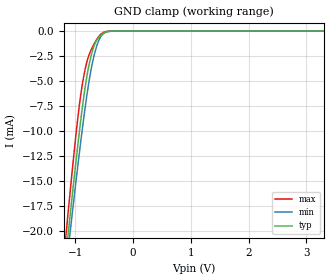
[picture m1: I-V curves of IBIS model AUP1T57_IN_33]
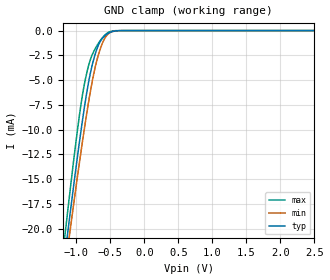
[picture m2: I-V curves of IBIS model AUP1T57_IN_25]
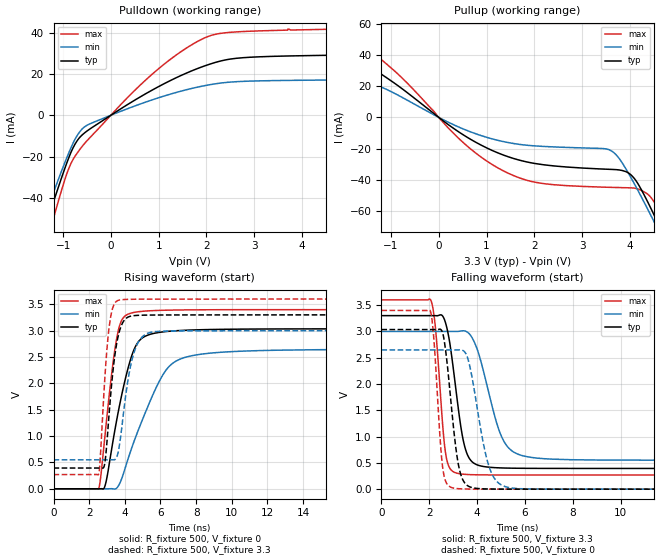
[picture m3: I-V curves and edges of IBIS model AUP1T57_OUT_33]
| TEXAS INSTRUMENTS INCORPORATED
| Standard Linear and Logic Group
| IBIS Model of SN74AUP1T57
| SINGLE-SUPPLY VOLTAGE TRANSLATER
| This file contains package information for the following:
|  SOT 6-pin (DBV) package as [Component] AUP1T57_DBV
|  SOT 6-pin (DCK) package as [Component] AUP1T57
|  DSBGA 6-pin (YEP_YZP) package as [Component] AUP1T57_YEP_YZP
| This device can be powered at the following Vccs:
|  3.3 volt Vcc
|  2.5 volt Vcc
| This file provides unique models under the [Model Selector] for each Vcc.
| For operation at a specific Vcc, select the appropriate model after each
| [Model Selector] keyword.
[IBIS Ver]   3.2
[Comment char]  |_char
[File Name]   sn74aup1t57.ibs
[File Rev]   1.1 | x_die
[Date]   July 14, 2004
[Source]   Data created from TI-SPICE simulations at TI-SLL.
[Notes]   The following is an IBIS list for the AUP1T57.
   Please contact sllibis@ti.com with questions and
   comments concerning SLL IBIS models.
   - FILE REV HISTORY
   - 1.1 Release IBIS file on 10/01/04
   - Non-monotonic data in pullup due to special output circuit.
   - Power clamp data deleted as there is no power-clamp diode.
   - YEP and YZP packages are package preview only at this date.
[Disclaimer] Property of Texas Instruments Incorporated.  Unauthorized
   reproduction and/or distribution is strictly prohibited.
   This product is protected under copyright law.
   Created  2004, (C) Copyright  2004, Texas Instruments
   Incorporated, All Rights Reserved
   UNLESS THERE IS A SIGNED, WRITTEN AGREEMENT TO THE
   CONTRARY, TEXAS INSTRUMENTS (TI) IS PROVIDING THE IBIS
   MODELS  AND WITHOUT ANY WARRANTY, EXPRESSED OR
   IMPLIED.  TI assumes no liability for:
   1) the accuracy of the IBIS models provided to your
   company;
   2) the proper functioning of these IBIS Models in your
   design or for any resulting applications; or
   3) infringement of patents, copyrights or intellectual
   property rights resulting from your use of these IBIS
   models.
   TI provides IBIS Models as a service to our customers.
   You and your company shall not distribute, sell or give
   these models to anyone else without prior written
   permission from TI.
   TI reserves the right to make changes to our products or
   to discontinue any semiconductor product or service
   without notice, and advises our customers to obtain the
   latest version of relevant information to verify, before
   placing orders, that the information being relied on is
   current.
   Please be aware that your receipt and use of the IBIS
   information provided shall serve as acceptance of these
   terms and conditions.  If you do not accept these terms,
   you should return or destroy the IBIS models and any
   other accompanying information immediately.
| Component AUP1T57_DBV 6-pin SOT
[Component]   AUP1T57_DBV
[Manufacturer]   Texas Instruments, Inc.
[Package]
|   typ   min   max
R_pkg   2.500e-02   1.900e-02   3.700e-02
L_pkg   1.524e-09   1.260e-09   1.751e-09
C_pkg   2.450e-13   1.980e-13   2.640e-13
[Pin]   signal_name   model_name   R_pin   L_pin   C_pin
1   B   AUP1T57_IN   2.100e-02   1.405e-09   2.460e-13
2   GND   GND   3.700e-02   1.751e-09   2.630e-13
3   A   AUP1T57_IN   2.600e-02   1.493e-09   2.470e-13
4   Y   AUP1T57_IN   1.900e-02   1.620e-09   2.640e-13
5   VCC   POWER   2.400e-02   1.260e-09   1.980e-13
6   C   AUP1T57_OUT   2.100e-02   1.617e-09   2.500e-13
| Component AUP1T57_DCK 6-pin SOT
[Component]   AUP1T57_DCK
[Manufacturer]   Texas Instruments, Inc.
[Package]
|   typ   min   max
R_pkg   1.400e-02   1.100e-02   2.100e-02
L_pkg   9.480e-10   7.840e-10   1.103e-09
C_pkg   1.910e-13   1.670e-13   2.050e-13
[Pin]   signal_name   model_name   R_pin   L_pin   C_pin
1   B   AUP1T57_IN   1.300e-02   9.840e-10   1.960e-13
2   GND   GND   2.100e-02   1.103e-09   2.050e-13
3   A   AUP1T57_IN   1.100e-02   9.980e-10   1.970e-13
4   Y   AUP1T57_IN   1.300e-02   9.040e-10   1.900e-13
5   VCC   POWER   1.500e-02   7.840e-10   1.670e-13
6   C   AUP1T57_OUT   1.200e-02   9.160e-10   1.950e-13
| Component AUP1T57_YEP_YZP 6-pin DSBGA
[Component]   AUP1T57_YEP_YZP
[Manufacturer]   Texas Instruments, Inc.
[Package]
|   typ   min   max
R_pkg   1.000e-03   1.000e-03   2.100e-02
L_pkg   2.450e-11   2.400e-11   1.103e-09
C_pkg   5.600e-14   0.000e+00   2.050e-13
[Pin]   signal_name   model_name   R_pin   L_pin   C_pin
1   B   AUP1T57_IN   1.000e-03   2.500e-11   6.400e-14
2   GND   GND   1.000e-03   2.400e-11   6.700e-14
3   A   AUP1T57_IN   1.000e-03   2.500e-11   6.400e-14
4   Y   AUP1T57_OUT   1.000e-03   2.500e-11   6.400e-14
5   VCC   POWER   1.000e-03   2.400e-11   6.700e-14
6   C   AUP1T57_IN   1.000e-03   2.500e-11   6.400e-14
| Model AUP1T57_IN
[Model Selector]   AUP1T57_IN
AUP1T57_IN_33   3.3 volt Vcc
AUP1T57_IN_25   2.5 volt Vcc
| Model AUP1T57_OUT
[Model Selector]   AUP1T57_OUT
AUP1T57_OUT_33   3.3 volt Vcc
AUP1T57_OUT_25   2.5 volt Vcc
| Models and submodels in the file (4): AUP1T57_IN_33 (Input), AUP1T57_IN_25 (Input), AUP1T57_OUT_33 (Output), AUP1T57_OUT_25 (Output)
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[Model]   AUP1T57_IN_33
Model_type  Input
Vinl=0.9
Vinh=2.1
| variable   typ   min   max
C_comp   1.41pF   1.16pF   1.79pF
[Temperature Range]   40   100   -40
| Ambient temperature   25   85   -40
[Voltage range]   3.3   3   3.6
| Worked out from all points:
|   GND clamp passes 1 mA (typ) near -0.64 V on its own axis
[GND Clamp]
| AUP1T57_IN_33
|   Voltage   I(typ)   I(min)   I(max)
-3.6V     -171.6mA   -163.5mA   -181.1mA
-1.16V    -22.22mA   -23.69mA   -20.18mA
-1.11V    -19.45mA   -21.09mA   -17.19mA
-1.085V   -18.08mA   -19.81mA   -15.71mA
-940mV    -10.5mA    -12.6mA    -7.822mA
-890mV    -8.117mA   -10.26mA   -5.698mA
-835mV    -5.768mA   -7.825mA   -3.925mA
-755mV    -3.153mA   -4.717mA   -2.255mA
-675mV    -1.463mA   -2.419mA   -1.277mA
-595mV    -617.7uA   -945.8uA   -546.7uA
-515mV    -215.4uA   -248.8uA   -134.4uA
3.3V      132.2pA    540.4pA    36.28pA
[Model]   AUP1T57_IN_25
Model_type  Input
Vinl=0.7
Vinh=1.6
| variable   typ   min   max
C_comp   1.46pF   1.21pF   1.77pF
[Temperature Range]   40   100   -40
| Ambient temperature   25   85   -40
[Voltage range]   2.5   2.3   2.7
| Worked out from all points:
|   GND clamp passes 1 mA (typ) near -0.64 V on its own axis
[GND Clamp]
| AUP1T57_IN_25
|   Voltage   I(typ)   I(min)   I(max)
-3.6V     -171.6mA   -163.5mA   -181.1mA
-1.165V   -22.5mA    -23.95mA   -20.48mA
-1.115V   -19.72mA   -21.35mA   -17.49mA
-1.09V    -18.36mA   -20.06mA   -16.01mA
-945mV    -10.75mA   -12.84mA   -8.061mA
-890mV    -8.117mA   -10.26mA   -5.698mA
-835mV    -5.768mA   -7.825mA   -3.925mA
-760mV    -3.287mA   -4.89mA    -2.329mA
-675mV    -1.463mA   -2.419mA   -1.277mA
-595mV    -617.7uA   -945.8uA   -546.7uA
-520mV    -233.1uA   -272.6uA   -149.9uA
2.5V      104.3pA    491.9pA    26.71pA
[Model]   AUP1T57_OUT_33
Model_type  Output
Vref =   0
Rref =   1E6
Cref =   30p
Vmeas =   1.65
| variable   typ   min   max
C_comp   2.73pF   1.81pF   4.12pF
| C_pullup   3.12pF   1.81pF   4.12pF
| C_pulldown   2.33pF   2.13pF   2.90pF
[Temperature Range]   40   100   -40
| Ambient temperature   25   85   -40
[Voltage range]   3.3   3   3.6
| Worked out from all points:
|   slope of the pulldown table from 0 to 0.495 V, typ, clamps not added: 68.4 ohm
|   slope of the pullup table from 0 to 0.495 V, typ, clamps not added: 45.8 ohm
|   rising waveform, R_fixture 500, V_fixture 0: 20-80 % time 1.11ns typ, 1.91ns min, 689ps max; typ from 0 V to 3.04 V
|   falling waveform, R_fixture 500, V_fixture 3.3: 20-80 % time 523ps typ, 877ps min, 330ps max; typ from 3.3 V to 0.394 V
|   rising waveform, R_fixture 500, V_fixture 3.3: 20-80 % time 506ps typ, 666ps min, 393ps max; typ from 0.394 V to 3.3 V
|   falling waveform, R_fixture 500, V_fixture 0: 20-80 % time 428ps typ, 642ps min, 287ps max; typ from 3.04 V to 0 V
[Pulldown]
| AUP1T57_OUT_33
|   Voltage   I(typ)   I(min)   I(max)
-3.6V     -218.7mA   -196.3mA   -248.6mA
-1.515V   -64.37mA   -57.31mA   -75.82mA
-1.39V    -55.35mA   -49.29mA   -65.41mA
-1.275V   -47.14mA   -42mA      -55.89mA
-870mV    -19.93mA   -17.62mA   -25.18mA
-720mV    -12.85mA   -10.38mA   -18.82mA
-545mV    -8.444mA   -5.509mA   -13.51mA
940mV     13.13mA    8.018mA    21.36mA
1.5V      19.56mA    11.86mA    31.27mA
2.045V    24.53mA    14.67mA    38.2mA
3.1V      28.27mA    16.63mA    40.81mA
7.2V      29.73mA    17.36mA    42.67mA
[Pullup]
| AUP1T57_OUT_33
|   Voltage   I(typ)   I(min)   I(max)
-3.6V     42.88mA    27.27mA    57.92mA
-2.465V   31.53mA    19.52mA    45.85mA
-1.53V    32.87mA    22.09mA    44.95mA
-755mV    18.1mA     12.64mA    24.89mA
555mV     -11.98mA   -7.942mA   -17.3mA
1.65V     -27.07mA   -17.13mA   -38.31mA
3.61V     -33.32mA   -21.39mA   -44.82mA
4.08V     -38.63mA   -41.77mA   -45.28mA
4.375V    -54.25mA   -58.9mA    -49.24mA
4.565V    -66.24mA   -70.37mA   -57.33mA
4.775V    -80.02mA   -83.29mA   -71.37mA
7.2V      -250.7mA   -240.9mA   -257mA
[Ramp]
| AUP1T57_OUT_33
| variable   typ   min   max
dV/dt_r   1.82/1.11E-09   1.59/1.92E-09   2.04/6.91E-10
dV/dt_f   1.75/5.32E-10   1.48/8.84E-10   2.01/3.34E-10
R_load = 500
[Rising Waveform]
| AUP1T57_OUT_33
R_fixture =   500
C_fixture =   0
L_fixture =   0
V_fixture =   0
V_fixture_min = 0
V_fixture_max = 0
|   Time   V(typ)   V(min)   V(max)
0s        24.73nV    82.54nV    2.123nV
2.535ns   -69.78uV   466.3nV    3.177mV
2.915ns   87.17mV    -39.41uV   1.104V
3.53ns    1.278V     8.769mV    2.828V
3.815ns   1.765V     183.7mV    3.191V
4.28ns    2.408V     668.6mV    3.326V
4.885ns   2.836V     1.224V     3.364V
6.145ns   2.977V     2.168V     3.387V
7.64ns    3.012V     2.517V     3.395V
29.99ns   3.035V     2.647V     3.399V
[Falling Waveform]
| AUP1T57_OUT_33
R_fixture =   500
C_fixture =   0
L_fixture =   0
V_fixture =   3.3
V_fixture_min = 3
V_fixture_max = 3.6
|   Time   V(typ)   V(min)   V(max)
0s        3.3V       3V         3.6V
2.075ns   3.3V       3V         3.585V
2.265ns   3.299V     3V         3.045V
2.68ns    3.166V     3V         698.3mV
3.16ns    1.735V     2.999V     303.1mV
3.455ns   864mV      3.011V     283.3mV
3.78ns    526.1mV    2.89V      275.4mV
5.035ns   403.5mV    989.8mV    269.8mV
6.06ns    396.4mV    619.8mV    269.4mV
29.99ns   394.1mV    550mV      269.3mV
[Rising Waveform]
| AUP1T57_OUT_33
R_fixture =   500
C_fixture =   0
L_fixture =   0
V_fixture =   3.3
V_fixture_min = 3
V_fixture_max = 3.6
|   Time   V(typ)   V(min)   V(max)
0s        394.1mV    550mV      269.3mV
2.53ns    394mV      550mV      274.2mV
2.63ns    394.8mV    550mV      625.7mV
2.865ns   462.5mV    550mV      2.023V
3.09ns    1.298V     550.4mV    2.979V
3.36ns    2.313V     549.7mV    3.468V
3.63ns    2.901V     698.2mV    3.575V
4.44ns    3.283V     2.498V     3.596V
5.425ns   3.296V     2.966V     3.599V
29.99ns   3.3V       3V         3.6V
[Falling Waveform]
| AUP1T57_OUT_33
R_fixture =   500
C_fixture =   0
L_fixture =   0
V_fixture =   0
V_fixture_min = 0
V_fixture_max = 0
|   Time   V(typ)   V(min)   V(max)
0s        3.035V     2.647V     3.399V
2.05ns    3.035V     2.647V     3.383V
2.195ns   3.035V     2.647V     2.847V
2.56ns    2.973V     2.647V     422.2mV
2.985ns   1.308V     2.647V     23.72mV
3.225ns   456.6mV    2.649V     9.221mV
3.49ns    115.3mV    2.606V     3.845mV
4.49ns    3.321mV    446.9mV    216.4uV
5.295ns   519.1uV    34.07mV    36.38uV
29.99ns   -4.172nV   156nV      -13.8nV
